FUNCTION_BLOCK Example12_DImacro //4x3 flyways 1 xbot - send digital signal to PMC, macro trigger from DI
VAR_INPUT
	Execute : BOOL;
END_VAR
VAR_OUTPUT
	Done : BOOL;
END_VAR
VAR_IN_OUT
	PM_Controller : PMControllerType;	// the planar motor controller to use
END_VAR
VAR
	PMC_XYMotion1 : PMC_XYMotion;
	PMC_ClearMacro1 : PMC_ClearMacro;
	PMC_XYMotion2 : PMC_XYMotion;
	PMC_XYMotion3 : PMC_XYMotion;
	PMC_SaveMacro1 : PMC_SaveMacro;
	DI_ID_array22 : ARRAY[0..21] OF USINT;
	macro_ID_array22 : ARRAY[0..21] OF USINT;
	xbotID_array22 : ARRAY[0..21] OF USINT;
	PMC_ConfigDI2RunMacro1 : PMC_ConfigDI2RunMacro;
	PMC_SendDigitalSignalToPMC1 : PMC_SendDigitalSignalToPMC;
	Delay1 : Delay;
	PMC_SendDigitalSignalToPMC2 : PMC_SendDigitalSignalToPMC;
END_VAR

//4x3 flyways 1 xbot - send digital signal to PMC, macro trigger from DI

//move xbot 1 to 60,60
PMC_XYMotion1(Execute := Execute,cmdLB := 1,XbotID := 1,Mode := 0,Type_ := 0,PosX := 0.06,PosY := 0.06,EndVel := 0,MaxVel := 1,MaxAcc := 10,PM_Controller := PM_Controller);

//clear macro 128
PMC_ClearMacro1(Execute := PMC_XYMotion1.Done,MacroID := 128,PM_Controller := PM_Controller);

//write move to 900,60 to macro 128
PMC_XYMotion2(Execute := PMC_ClearMacro1.Done,cmdLB := 3,XbotID := 128,Mode := 0,Type_ := 0,PosX := 0.9,PosY := 0.06,EndVel := 0,MaxVel := 1,MaxAcc := 10,PM_Controller := PM_Controller);

//write move to 900,660 to macro 128
PMC_XYMotion3(Execute := PMC_XYMotion2.Done,cmdLB := 4,XbotID := 128,Mode := 0,Type_ := 0,PosX := 0.9,PosY := 0.66,EndVel := 0,MaxVel := 1,MaxAcc := 10,PM_Controller := PM_Controller);

//save macro 128
PMC_SaveMacro1(Execute := PMC_XYMotion3.Done,MacroID := 128,PM_Controller := PM_Controller);

//set digital input 1 to trigger macro 128 on xbot 1
DI_ID_array22[0] := 1;
macro_ID_array22[0] := 128;
xbotID_array22[0] := 1;
PMC_ConfigDI2RunMacro1(Execute := PMC_SaveMacro1.Done,nDI := 1,DiID := DI_ID_array22,MacroID := macro_ID_array22,XbotID := xbotID_array22,PM_Controller := PM_Controller);

//set DI 1 to 0
PMC_SendDigitalSignalToPMC1(Enable := PMC_ConfigDI2RunMacro1.Done,DoID := 1,Level := FALSE,PM_Controller := PM_Controller);

Delay1(Execute := PMC_SendDigitalSignalToPMC1.Valid,Cycles := 1);

//set DI 1 to 1
PMC_SendDigitalSignalToPMC2(Enable := Delay1.Done,DoID := 1,Level := TRUE,PM_Controller := PM_Controller);

Done := PMC_SendDigitalSignalToPMC2.Valid;

END_FUNCTION_BLOCK
